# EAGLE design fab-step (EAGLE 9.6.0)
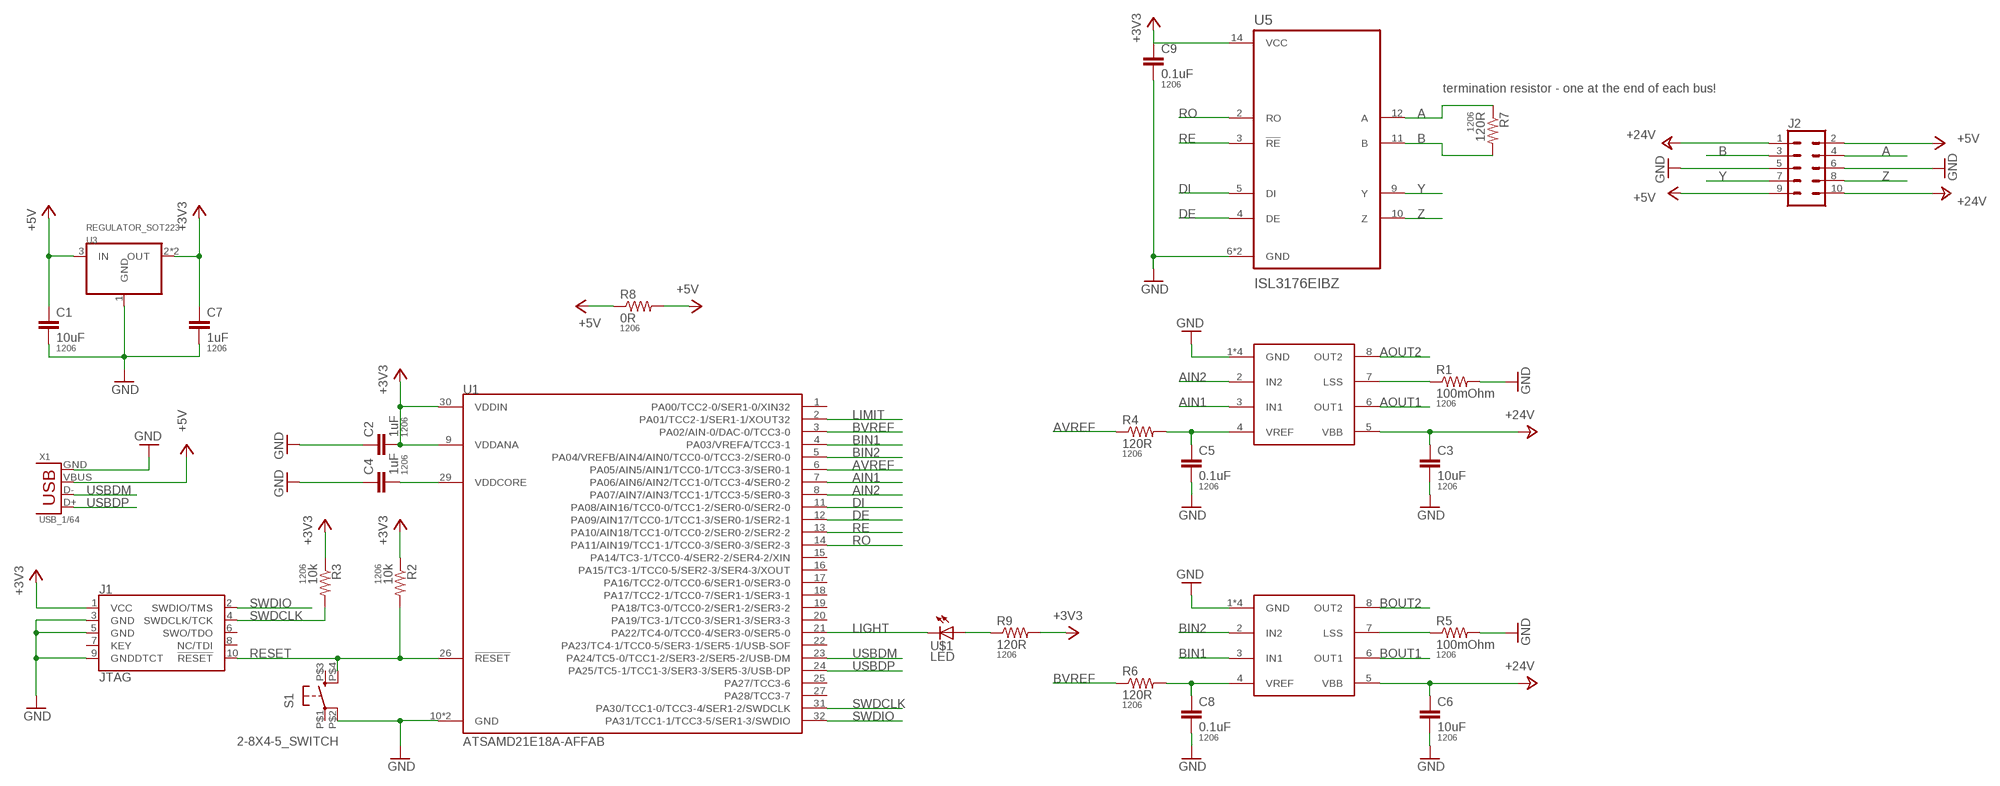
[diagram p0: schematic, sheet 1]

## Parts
C1  10uF  CAP1206  [1206]
C2  1uF  CAP1206  [1206]
C3  10uF  CAP1206  [1206]
C4  1uF  CAP1206  [1206]
C5  0.1uF  CAP1206  [1206]
C6  10uF  CAP1206  [1206]
C7  1uF  CAP1206  [1206]
C8  0.1uF  CAP1206  [1206]
C9  0.1uF  CAP1206  [1206]
J1  JTAG  CORTEX_JTAG_DEBUG_SMD  [2X5-SMD-1.27MM]
J2  CONN_05X2SMD_LONGPADS  [2X5-SHROUDED_SMD_LONGPADS]
R1  100mOhm  RESISTOR1206  [1206]
R2  10k  RESISTOR1206  [1206]
R3  10k  RESISTOR1206  [1206]
R4  120R  RESISTOR1206  [1206]
R5  100mOhm  RESISTOR1206  [1206]
R6  120R  RESISTOR1206  [1206]
R7  120R  RESISTOR1206  [1206]
R8  0R  RESISTOR1206  [1206]
R9  120R  RESISTOR1206  [1206]
S1  2-8X4-5_SWITCH  [TACT-SWITCH-KMR6]
U1  ATSAMD21E18A-AFFAB  [TQFP-32-FAB]
U2  A4950FAB  [SOIC8_PAD_THRU_FAB]
U3  REGULATOR_SOT223  [SOT223]
U4  A4950FAB  [SOIC8_PAD_THRU_FAB]
U5  ISL3176EIBZ  [SOIC-14]
U$1  LED  [LED1206]
X1  USB_1/64  [DX4R005HJ5_64]

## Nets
+3V3: C2.2 C7.1 C9.1 J1.1(VCC) R2.1 R3.1 R9.2 U1.9(VDDANA) U1.30(VDDIN) U3.2(OUT) U3.4(OUT) U5.14(VCC)
+5V: C1.1 J2.2 J2.9 R8.1 R8.2 U3.3(IN) X1.VBUS
+24V: C3.1 C6.1 J2.1 J2.10 U2.5(VBB) U4.5(VBB)
A: J2.4 R7.1 U5.12(A)
AIN1: U1.7(PA06/AIN6/AIN2/TCC1-0/TCC3-4/SER0-2) U2.3(IN1)
AIN2: U1.8(PA07/AIN7/AIN3/TCC1-1/TCC3-5/SER0-3) U2.2(IN2)
AOUT1: U2.6(OUT1)
AOUT2: U2.8(OUT2)
AVREF: R4.1 U1.6(PA05/AIN5/AIN1/TCC0-1/TCC3-3/SER0-1)
B: J2.3 R7.2 U5.11(B)
BIN1: U1.4(PA03/VREFA/TCC3-1) U4.3(IN1)
BIN2: U1.5(PA04/VREFB/AIN4/AIN0/TCC0-0/TCC3-2/SER0-0) U4.2(IN2)
BOUT1: U4.6(OUT1)
BOUT2: U4.8(OUT2)
BVREF: R6.1 U1.3(PA02/AIN-0/DAC-0/TCC3-0)
DE: U1.12(PA09/AIN17/TCC0-1/TCC1-3/SER0-1/SER2-1) U5.4(DE)
DI: U1.11(PA08/AIN16/TCC0-0/TCC1-2/SER0-0/SER2-0) U5.5(DI)
GND: C1.2 C2.1 C3.2 C4.1 C5.2 C6.2 C7.2 C8.2 C9.2 J1.3(GND) J1.5(GND) J1.9(GNDDTCT) J2.5 J2.6 R1.2 R5.2 S1.P$2(P1) U1.10(GND) U1.28(GND) U2.1(GND) U2.P$1(GND) U2.P$2(GND) U2.P$3(GND) U3.1(GND) U4.1(GND) U4.P$1(GND) U4.P$2(GND) U4.P$3(GND) U5.6(GND) U5.7(GND) X1.GND
LIGHT: U1.21(PA22/TC4-0/TCC0-4/SER3-0/SER5-0) U$1.2(C)
LIMIT: U1.2(PA01/TCC2-1/SER1-1/XOUT32)
N$1: C4.2 U1.29(VDDCORE)
N$2: R1.1 U2.7(LSS)
N$3: C5.1 R4.2 U2.4(VREF)
N$4: R5.1 U4.7(LSS)
N$5: C8.1 R6.2 U4.4(VREF)
N$7: R9.1 U$1.1(A)
RE: U1.13(PA10/AIN18/TCC1-0/TCC0-2/SER0-2/SER2-2) U5.3(!RE)
RESET: J1.10(!RESET) R2.2 S1.P$4(S1) U1.26(!RESET)
RO: U1.14(PA11/AIN19/TCC1-1/TCC0-3/SER0-3/SER2-3) U5.2(RO)
SWDCLK: J1.4(SWDCLK/TCK) R3.2 U1.31(PA30/TCC1-0/TCC3-4/SER1-2/SWDCLK)
SWDIO: J1.2(SWDIO/TMS) U1.32(PA31/TCC1-1/TCC3-5/SER1-3/SWDIO)
USBDM: U1.23(PA24/TC5-0/TCC1-2/SER3-2/SER5-2/USB-DM) X1.D-
USBDP: U1.24(PA25/TC5-1/TCC1-3/SER3-3/SER5-3/USB-DP) X1.D+
Y: J2.7 U5.9(Y)
Z: J2.8 U5.10(Z)
Unconnected: J1.6(SWO/TDO) J1.7(KEY) J1.8(NC/TDI) S1.P$1(P) S1.P$3(S) U1.1(PA00/TCC2-0/SER1-0/XIN32) U1.15(PA14/TC3-1/TCC0-4/SER2-2/SER4-2/XIN) U1.16(PA15/TC3-1/TCC0-5/SER2-3/SER4-3/XOUT) U1.17(PA16/TCC2-0/TCC0-6/SER1-0/SER3-0) U1.18(PA17/TCC2-1/TCC0-7/SER1-1/SER3-1) U1.19(PA18/TC3-0/TCC0-2/SER1-2/SER3-2) U1.20(PA19/TC3-1/TCC0-3/SER1-3/SER3-3) U1.22(PA23/TC4-1/TCC0-5/SER3-1/SER5-1/USB-SOF) U1.25(PA27/TCC3-6) U1.27(PA28/TCC3-7)

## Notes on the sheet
- termination resistor - one at the end of each bus!

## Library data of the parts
C1-C9 = passives:CAP: Capacitor; PACKAGE: 1206
J1 = SparkFun-Connectors:CORTEX_JTAG_DEBUG: Cortex Debug Connector - 10 pin Supports JTAG debug, Serial Wire debug, and Serial Wire Viewer. PTH and SMD connector options available. General Connector Information Products: PTH Connector -via Digi-Key SparkFun PSoc SparkFun T; PROD_ID: CONN-14503
J2 = SparkFun-Connectors:CONN_05X2: Multi connection point. Often used as Generic Header-pin footprint for 0.1 inch spaced/style header connections For AVR SPI programming port, see special device with nice symbol: "AVR_SPI_PROG_5x2.dev" You can populate with any combo of single row headers, but if you'd like an exact match, check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
R1-R9 = passives:RESISTOR: Resistor; PACKAGE: 1206
S1 = passives:2-8X4-5_SWITCH
U1 = microcontrollers:ATSAMD21E18A-AF: The SAM D21 is a series of low-power microcontrollers using the 32-bit ARM® Cortex® -M0+ processor, and ranging from 32- to 64-pins with up to 256KB Flash and 32KB of SRAM. The SAM D21 operate at a maximum frequency of 48MHz and reach 2.46 CoreMark® /MHz. Check prices
U2 U4 = power:A4950
U3 = power:REGULATOR_SOT223
U5 = comm:ISL3176EIBZ
U$1 = fablab:LED: LED
X1 = connector:USB: SMD micro USB connector as found in the fablab inventory. Three footprint variants included: 609-4613-1-ND used by Jake original, as described by manufacturer's datasheet for milling with the 1/100" bit for milling with the 1/64" bit Made by Zaerc.

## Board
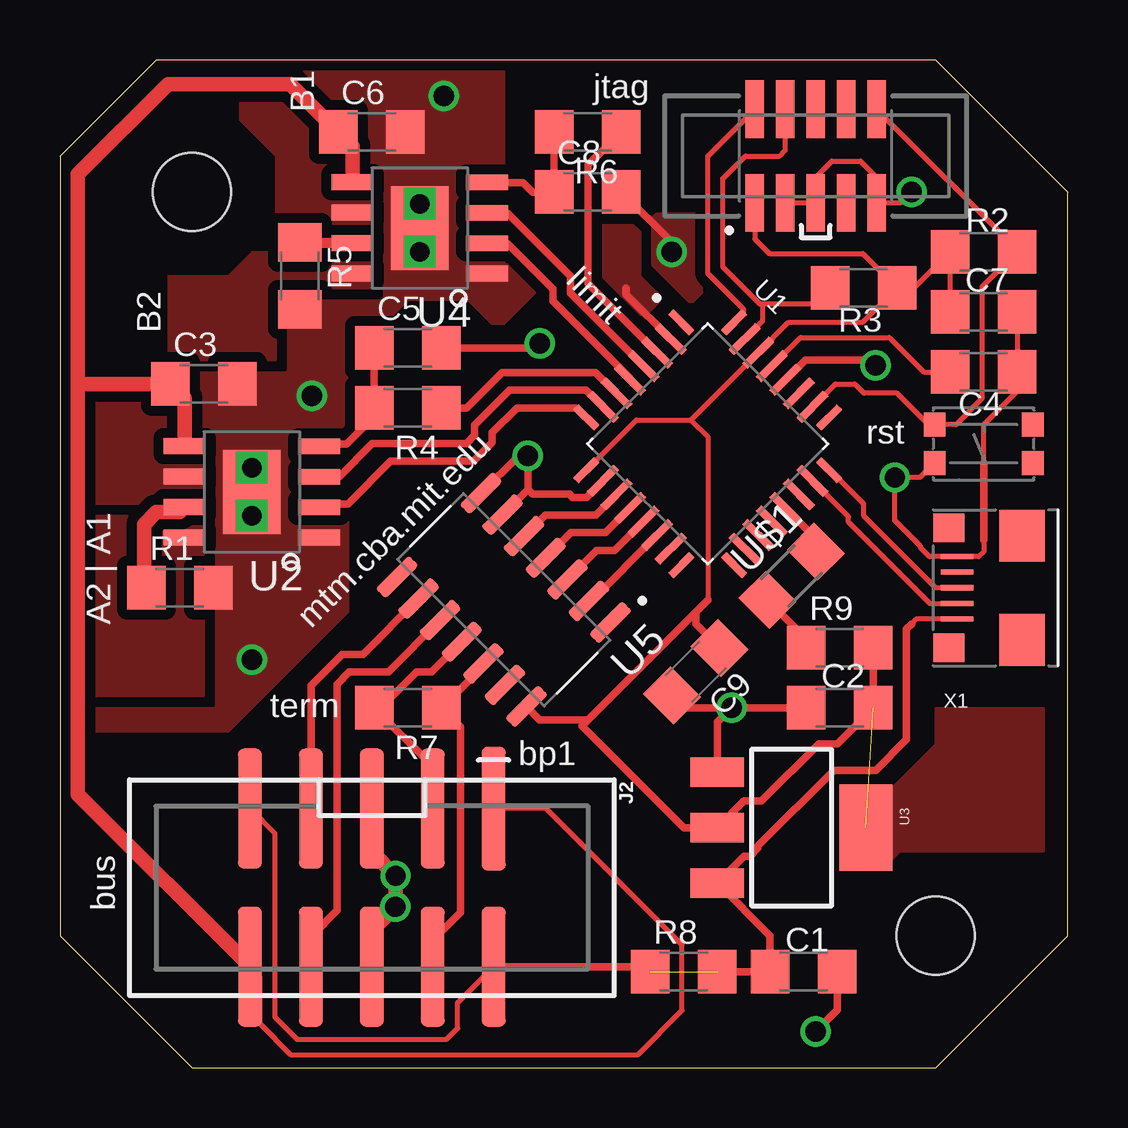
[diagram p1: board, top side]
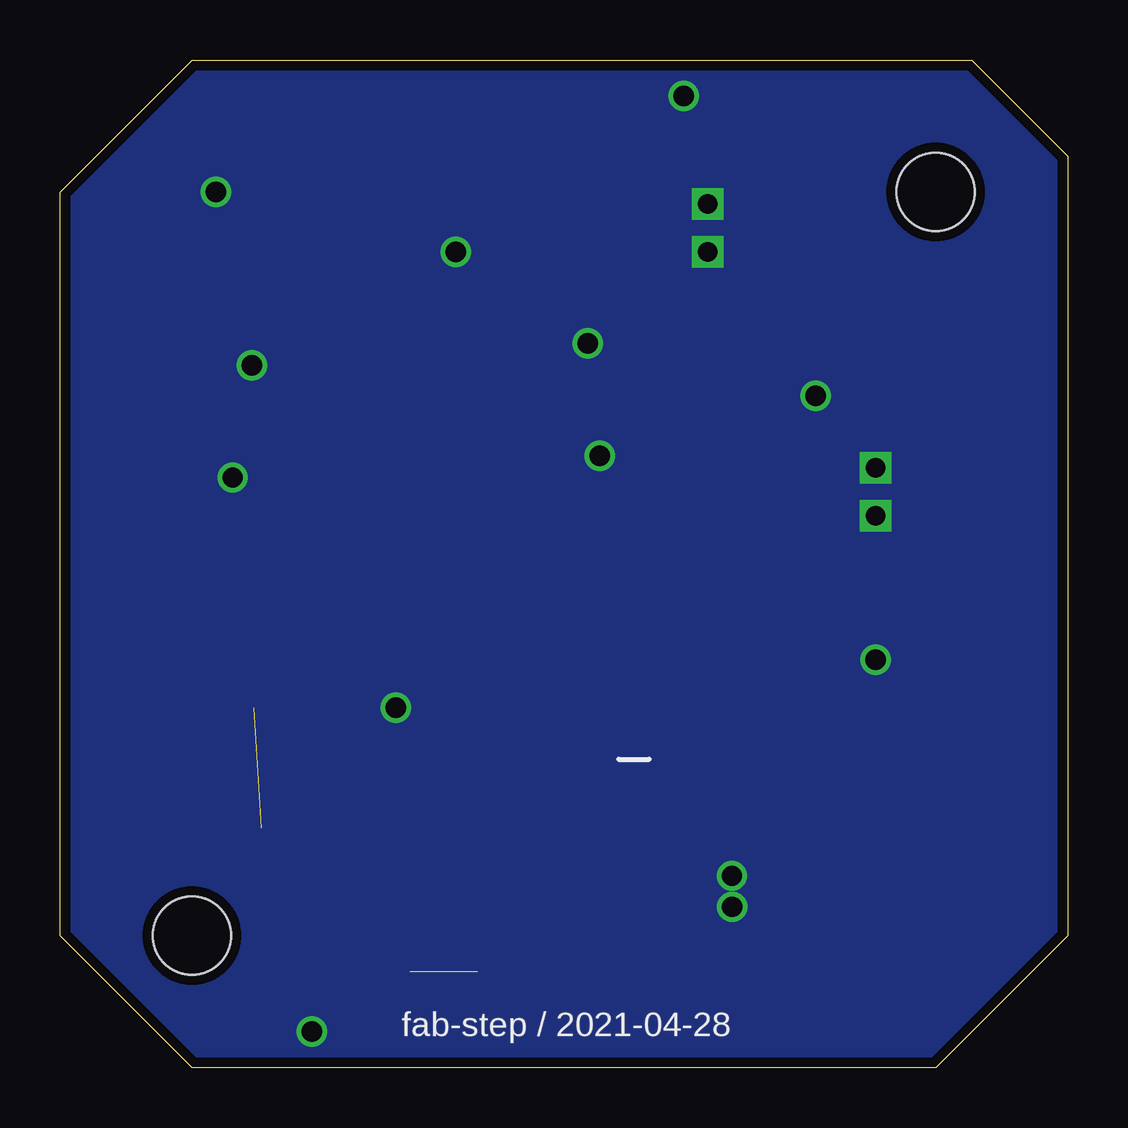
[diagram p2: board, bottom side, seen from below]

Size 42 x 42 mm. Coordinates in mm from the lower left corner, seen from the top.
Outline: 5.5,0 36.5,0 42,5.5 42,36.5 36.5,42 4,42 0,38 0,5.5 5.5,0
Copper layers (1*16): Top 0.035mm / dielectric 1.5mm / Bottom 0.035mm
Design rules "default *": minimum track width 8mil, minimum drill 33mil, track to track 17mil, track to pad 17mil, pad to pad 17mil, via to via 17mil, smd to smd 6mil, copper to edge 17mil, drill to drill 6mil, minimum pad ring 10mil, minimum via ring 8mil, stop-mask expansion 4mil, vias tented up to drill 35mil, thermal gap 17mil
Holes 3.25 mm at 36.5,5.5 5.5,36.5

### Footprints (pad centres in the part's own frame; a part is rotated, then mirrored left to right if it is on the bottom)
1206 = smd 1.6 x 1.8: 1 -1.4,0; 2 1.4,0
2X5-SMD-1.27MM = smd 0.76 x 2.4: 1 2.54,1.95; 2 2.54,-1.95; 3 1.27,1.95; 4 1.27,-1.95; 5 0,1.95; 6 0,-1.95; 7 -1.27,1.95; 8 -1.27,-1.95; 9 -2.54,1.95; 10 -2.54,-1.95
2X5-SHROUDED_SMD_LONGPADS = smd 5.15 x 1: 1 -3.294,5.08 | smd 5 x 1: 2 3.294,5.08; 3 -3.294,2.54; 4 3.294,2.54; 5 -3.294,0; 6 3.294,0; 7 -3.294,-2.54; 8 3.294,-2.54; 9 -3.294,-5.08; 10 3.294,-5.08
TACT-SWITCH-KMR6 = smd 0.9 x 1: P$1 -2.05,0.8; P$2 2.05,0.8; P$3 -2.05,-0.8; P$4 2.05,-0.8
TQFP-32-FAB = smd 1.25 x 0.35: 1 -4.355,2.8; 8 -4.355,-2.8; 17 4.355,-2.8; 24 4.355,2.8 | smd 1.6 x 0.35: 2 -4.18,2; 3 -4.18,1.2; 4 -4.18,0.4; 5 -4.18,-0.4; 6 -4.18,-1.2; 7 -4.18,-2; 18 4.18,-2; 19 4.18,-1.2; 20 4.18,-0.4; 21 4.18,0.4; 22 4.18,1.2; 23 4.18,2 | smd 0.35 x 1.25: 9 -2.8,-4.355; 16 2.8,-4.355; 25 2.8,4.355; 32 -2.8,4.355 | smd 0.35 x 1.6: 10 -2,-4.18; 11 -1.2,-4.18; 12 -0.4,-4.18; 13 0.4,-4.18; 14 1.2,-4.18; 15 2,-4.18; 26 2,4.18; 27 1.2,4.18; 28 0.4,4.18; 29 -0.4,4.18; 30 -1.2,4.18; 31 -2,4.18
SOIC8_PAD_THRU_FAB = smd 1.75 x 0.65: 1 -2.8,1.905; 2 -2.8,0.645; 3 -2.8,-0.625; 4 -2.8,-1.895; 5 2.8,-1.905; 6 2.8,-0.635; 7 2.8,0.635; 8 2.8,1.905 | smd 2.41 x 3.5: P$1 0,0 | drill 0.8 square: P$2 0,1; P$3 0,-1
SOT223 = smd 1.219 x 2.235: 1 -2.311,-3.099; 2 0,-3.099; 3 2.311,-3.099 | smd 3.6 x 2.2: 4 0,3.099
SOIC-14 = smd 1.97 x 0.6: 1 -2.475,3.81; 2 -2.475,2.54; 3 -2.475,1.27; 4 -2.475,0; 5 -2.475,-1.27; 6 -2.475,-2.54; 7 -2.475,-3.81; 8 2.475,-3.81; 9 2.475,-2.54; 10 2.475,-1.27; 11 2.475,0; 12 2.475,1.27; 13 2.475,2.54; 14 2.475,3.81
LED1206 = smd 1.6 x 1.803: 1 -1.422,0; 2 1.422,0
DX4R005HJ5_64 = smd 0.21 x 1.35: D+ 0,1.6; D- -0.65,1.6; GND 1.3,1.6; ID 0.65,1.6; VBUS -1.3,1.6 | smd 1.2 x 1.3: GND@1 -2.5,1.95; GND@2 2.5,1.95 | smd 2.15 x 1.9: GND@3 -2.175,-1.1; GND@4 2.175,-1.1

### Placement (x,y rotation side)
C1  31,4 0 top
C2  32.5,15 0 top
C3  6,28.5 0 top
C4  38.5,29 180 top
C5  14.5,30 0 top
C6  13,39 0 top
C7  38.5,31.5 0 top
C8  22,36.5 0 top
C9  26.5,16.5 225 top
J1  31.5,38 180 top
J2  13,7.5 270 top
R1  5,20 0 top
R2  38.5,34 0 top
R3  33.5,32.5 180 top
R4  14.5,27.5 180 top
R5  10,33 270 top
R6  22,39 180 top
R7  14.5,15 180 top
R8  26,4 0 top
R9  32.5,17.5 0 top
S1  38.5,26 180 top
U1  27,26 315 top
U2  8,24 180 top
U3  30.5,10 270 top
U4  15,35 180 top
U5  18.5,19.5 225 top
U$1  30.5,20.5 45 top
X1  39,20 90 top

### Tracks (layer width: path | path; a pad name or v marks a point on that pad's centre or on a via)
+3V3  (1 unrouted)
  Top 0.203: 26.3,27 U1.30 30.37,31.07 33.47,31.07 R3.1 | U1.9 24.04,27 26.3,27 | C7.1 R2.1 35.6,32.5 R3.1 | J1.1 28.96,34.54 29.57,33.93 33.47,33.93 R3.1 | 26.3,27 27,26.3 27,19.5
  Top 0.305: 27,19.5 26.5,19 | 26.5,19 22,14.5 | 22,14.5 21.75,14.25 26,10 U3.2 28.52,11.12 29.24,11.12 31.63,13.5 32.4,13.5 C2.2 R9.2 | U5.14 20,14.5 22,14.5 | 26.5,19 26.5,18.48 C9.1
  pour Top (rank 2): 33,11.5 34.5,11.5 36.5,13.5 36.5,15 41,15 41,9 35,9 34.5,8.5 33,8.5
+5V  (1 unrouted)
  Top 0.203: J2.9 8.95,9.76 8.95,2.1 9.89,1.17 16.11,1.17 16.57,1.63 16.57,2.7 J2.2 | X1.VBUS 35.7,18.7 35.5,18.5
  Top 0.305: J2.2 24.39,4.21 R8.1 | 35.5,18.5 35.28,18.28 35.28,13.67 34,12.38 32.26,12.38 29.1,9.23 29.1,9.15 28.76,8.81 28.52,8.81 U3.3 29.6,5.49 C1.1 R8.2
+24V
  Top 0.203: J2.10 8.06,4.06 8.32,3.81 8.32,1.84 9.62,0.54 24.09,0.54 25.93,2.38 25.93,5.12 20.26,10.79 J2.1
  Top 0.61: 8.06,4.06 0.74,11.39 0.74,28.5 | 0.74,28.5 0.74,37.24 4.5,41 9.6,41 C6.1 12.2,38.4 U4.5 | 0.74,28.5 C3.1 5.2,27.9 U2.5
A
  Top 0.305: U5.12 17.65,16.75 R7.1 16.7,14.2 16.7,6.46 15.54,5.3 J2.4
AIN1
  Top 0.305: U2.3 11.62,24.62 13.02,26.02 16.94,26.02 17.28,26.36 17.28,26.78 18.74,28.24 21.93,28.24 U1.7
AIN2
  Top 0.305: U2.2 10.95,23.5 12,23.5 13.78,25.28 17.25,25.28 18.02,26.05 18.02,26.48 19.04,27.5 21.5,27.5 21.9,27.1 U1.8
AOUT1
  pour Top (rank 2, no thermals): 6,23.5 1,23.5 1,28.5 6,28.5
AOUT2
  pour Top (no thermals): 6,23 1,23 1,15.5 6,15.5
AVREF
  Top 0.305: R4.1 16.96,27.5 18.43,28.97 22.33,28.97 U1.6
B
  Top 0.305: U5.11 15.48,16.48 14.86,16.48 13.37,15 R7.2 15.5,12.6 15.5,10.83 J2.3
BIN1
  Top 0.305: U4.3 18.65,35.62 21.28,33 21.28,32.29 U1.4
BIN2
  Top 0.305: U4.2 18.64,34.35 20.54,32.46 20.54,31.95 23.76,28.73 U1.5
BOUT1
  pour Top (no thermals): 13,35 9,35 9,38 7.5,39.5 7.5,40.5 10.5,40.5 13,38
BOUT2
  pour Top (no thermals): 13,34 8,34 7,33 4.5,33 4.5,29.5 9,29.5 9,32.5 13,32.5
BVREF
  Top 0.305: R6.1 22.38,37.98 22.36,37.98 22.02,37.64 22.02,32.68 U1.3
DE
  Top 0.305: U1.12 22.73,22.3 21.3,22.3 U5.4
DI
  Top 0.305: U1.11 22.34,23.03 20.24,23.03 U5.5
GND  (via drill 0.84)
  Top 0.203: C7.2 C4.1 39.9,28.2 38.5,26.8 38.5,25.2 | J1.3 J1.5 31.5,37.11 32.17,37.78 33.37,37.78 34.04,37.11 J1.9 35.05,36.05 v35.5,36.5 | 38.5,22 38.5,21.5 38.3,21.3 X1.GND 36.25,21.3 35.87,21.68 35.87,21.73 34.8,22.8 v34.8,24.6 35.85,24.6 S1.P$2
  Top 0.305: C2.1 v28,15 | U3.1 27.4,14.4 v28,15 | 38.5,22 38.5,25.2 | U1.28 31.07,29.5 33.77,29.5 v34,29.27 | U5.7 19.11,25.5 v19.5,25.5 19.5,24.09 | U5.6 19.5,24.09 | U1.10 21.94,23.77 21.36,23.77 21.23,23.9 19.69,23.9 19.5,24.09 | C5.2 19.81,30 v20,30.19 | C8.2 25.5,34.4 v25.5,34 | v28,15 26.02,15 C9.2 | C1.2 32.4,2.4 v31.5,1.5
  Top 0.61: J2.6 13,5.72 v13.98,6.7 13.99,6.71 v13.99,7.99 13,8.98 J2.5
  other vias: 16,40.5 10.5,28 8,17
  pour Top (rank 6, no thermals): 18.5,42.5 18.5,33.5 19,33.5 20,32.5 18.5,31 18,31 17,32 14.5,32 13.5,31 12,31 12,19 7,14 1,14 -0.5,15.5 -0.5,42.5
  pour Bottom (rank 2, no thermals): -0.5,43 42.5,43 42.5,-0.5 -0.5,-0.5
  pour Top: 24.9,35.5 24.8,35.4 24.8,33.7 24.8,33.5 26.3,32 27.1,32.8 26.9,33 26.9,33.7 26.9,35.1 26.6,35.4 26.5,35.5
LIGHT
  Top 0.305: U1.21 31.51,22.06 U$1.2
LIMIT
  Top 0.305: U1.2 23.6,32.23 23.6,32.5
  pour Top (rank 2): 22.5,35.2 22.5,32.9 23.3,32.1 23.9,31.5 24.4,31.5 25.1,32.2 25.1,32.7 25.1,34 24.4,34.7 23.9,35.2
N$1
  Top 0.203: U1.29 30.87,30.43 34.57,30.43 36,29 C4.2
N$2
  Top 0.61: U2.7 4.99,23.16 4.02,23.16 3.5,22.64 3.5,20.1 R1.1
N$3
  Top 0.305: U2.4 10.9,26 11.96,26 13.1,27.14 R4.2 C5.1
N$4
  Top 0.406: U4.7 10.04,34.37 R5.1
N$5
  Top 0.305: U4.4 19.3,36.9 19.7,36.5 C8.1 R6.2
N$7
  Top 0.305: U$1.1 31.1,17.89 R9.1
RE
  Top 0.305: U1.13 23.12,21.56 22.36,21.56 U5.3
RESET
  Top 0.203: J1.10 39.9,34.09 R2.2 38.43,32.53 38.43,27.88 37.35,26.8 S1.P$4 36.2,26.8 34.89,28.11 33.52,28.11 33.13,28.5 32.33,28.5 U1.26
RO
  Top 0.305: U1.14 22.15,19.45 U5.2
SWDCLK
  Top 0.203: J1.4 30.23,38.23 30,38 28.58,38 27.64,37.06 27.64,33.37 29.18,31.82 29.3,31.82 | R3.2 31.42,31.82 29.3,31.82 | U1.31 29.3,31.13 29.3,31.82
SWDIO
  Top 0.203: J1.2 27,37.99 27,33.1 28.5,31.6 28.5,31.46 U1.32
USBDM
  Top 0.203: X1.D- 36.25,19.35 32.87,22.74 32.87,22.96 U1.23
USBDP
  Top 0.203: X1.D+ 36.5,20 33.5,23 33.5,23.5 32.1,24.9 U1.24
Y
  Top 0.305: J2.7 10.46,15.93 11.75,17.22 12.63,17.22 U5.9
Z
  Top 0.305: U5.10 13.69,16.48 12.06,16.48 11.54,15.97 11.54,6.54 10.5,5.5 10.5,4.5 10.63,4.37 J2.8

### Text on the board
tPlace: B1 | jtag | B2 | limit | rst | mtm.cba.mit.edu | A2 | A1 | term | bp1 | bus
bPlace: fab-step / 2021-04-28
